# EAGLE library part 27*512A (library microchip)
CMOS EPROM 512 K (64 K x 8)
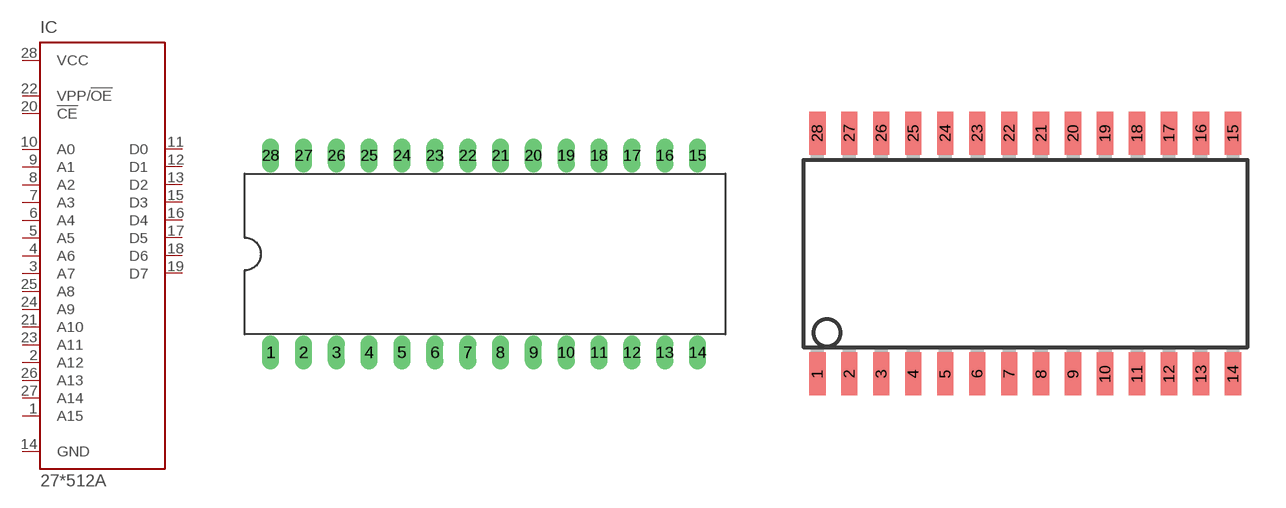
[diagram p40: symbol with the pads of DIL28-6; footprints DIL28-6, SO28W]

Designator prefix IC

## 27C512AP (MPN: M27C512-90B6; OC_FARNELL: 1642690; OC_NEWARK: 20M6389)  [DIL28-6]
1  A15  in
2  A12  in
3  A7  in
4  A6  in
5  A5  in
6  A4  in
7  A3  in
8  A2  in
9  A1  in
10  A0  in
11  D0  hiz
12  D1  hiz
13  D2  hiz
14  GND  pwr
15  D3  hiz
16  D4  hiz
17  D5  hiz
18  D6  hiz
19  D7  hiz
20  !CE  in
21  A10  in
22  VPP/!OE  in
23  A11  in
24  A9  in
25  A8  in
26  A13  in
27  A14  in
28  VCC  pwr

## 27C512ASO (OC_FARNELL: unknown; OC_NEWARK: unknown)  [SO28W]
Pads as for DIL28-6

## 27C512AL (MPN: M27C512-90C1; OC_FARNELL: 1218315; OC_NEWARK: 24M5090)  [PLCC-32]
2  A15  in
3  A12  in
4  A7  in
5  A6  in
6  A5  in
7  A4  in
8  A3  in
9  A2  in
10  A1  in
11  A0  in
13  D0  hiz
14  D1  hiz
15  D2  hiz
16  GND  pwr
18  D3  hiz
19  D4  hiz
20  D5  hiz
21  D6  hiz
22  D7  hiz
23  !CE  in
24  A10  in
25  VPP/!OE  in
27  A11  in
28  A9  in
29  A8  in
30  A13  in
31  A14  in
32  VCC  pwr

## 27C512ATS (OC_FARNELL: unknown; OC_NEWARK: unknown), 27LV512ATS (OC_FARNELL: unknown; OC_NEWARK: unknown)  [TSOP28]
1  VPP/!OE  in
2  A11  in
3  A9  in
4  A8  in
5  A13  in
6  A14  in
7  VCC  pwr
8  A15  in
9  A12  in
10  A7  in
11  A6  in
12  A5  in
13  A4  in
14  A3  in
15  A2  in
16  A1  in
17  A0  in
18  D0  hiz
19  D1  hiz
20  D2  hiz
21  GND  pwr
22  D3  hiz
23  D4  hiz
24  D5  hiz
25  D6  hiz
26  D7  hiz
27  !CE  in
28  A10  in

## 27512AVS (OC_FARNELL: unknown; OC_NEWARK: unknown)  [VSOP28-8X13]
Pads as for DIL28-6

## Footprint DIL28-6 (pad centres in mm)
Dual In Line package type P
drill 0.813 long: 1 -16.51,-7.62; 2 -13.97,-7.62; 3 -11.43,-7.62; 4 -8.89,-7.62; 5 -6.35,-7.62; 6 -3.81,-7.62; 7 -1.27,-7.62; 8 1.27,-7.62; 9 3.81,-7.62; 10 6.35,-7.62; 11 8.89,-7.62; 12 11.43,-7.62; 13 13.97,-7.62; 14 16.51,-7.62; 15 16.51,7.62; 16 13.97,7.62; 17 11.43,7.62; 18 8.89,7.62; 19 6.35,7.62; 20 3.81,7.62; 21 1.27,7.62; 22 -1.27,7.62; 23 -3.81,7.62; 24 -6.35,7.62; 25 -8.89,7.62; 26 -11.43,7.62; 27 -13.97,7.62; 28 -16.51,7.62

## Footprint SO28W (pad centres in mm)
28-Lead Plastic Small Outline (SO) Wide, 300 mil Body (SOIC) Source: http://ww1.microchip.com/downloads/en/devicedoc/39632c.pdf
smd 0.65 x 1.7: 1 -7.62,-4.78; 2 -6.35,-4.78; 3 -5.08,-4.78; 4 -3.81,-4.78; 5 -2.54,-4.78; 6 -1.27,-4.78; 7 0,-4.78; 8 1.27,-4.78; 9 2.54,-4.78; 10 3.81,-4.78; 11 5.08,-4.78; 12 6.35,-4.78; 13 7.62,-4.78; 14 8.89,-4.78; 15 8.89,4.78; 16 7.62,4.78; 17 6.35,4.78; 18 5.08,4.78; 19 3.81,4.78; 20 2.54,4.78; 21 1.27,4.78; 22 0,4.78; 23 -1.27,4.78; 24 -2.54,4.78; 25 -3.81,4.78; 26 -5.08,4.78; 27 -6.35,4.78; 28 -7.62,4.78

## Footprint PLCC-32 (pad centres in mm)
PLASTIC LEADED CHIP CARRIER rectangle, package type L
smd 2.2 x 0.6: 1 -6.83,0; 2 -6.83,-1.27; 3 -6.83,-2.54; 4 -6.83,-3.81; 14 6.83,-3.81; 15 6.83,-2.54; 16 6.83,-1.27; 17 6.83,0; 18 6.83,1.27; 19 6.83,2.54; 20 6.83,3.81; 30 -6.83,3.81; 31 -6.83,2.54; 32 -6.83,1.27
smd 0.6 x 2.2: 5 -5.08,-5.56; 6 -3.81,-5.56; 7 -2.54,-5.56; 8 -1.27,-5.56; 9 0,-5.56; 10 1.27,-5.56; 11 2.54,-5.56; 12 3.81,-5.56; 13 5.08,-5.56; 21 5.08,5.56; 22 3.81,5.56; 23 2.54,5.56; 24 1.27,5.56; 25 0,5.56; 26 -1.27,5.56; 27 -2.54,5.56; 28 -3.81,5.56; 29 -5.08,5.56

## Footprint TSOP28 (pad centres in mm)
Thin Small Outline Package Gull Wing type I, package type TS
smd 0.3 x 1: 1 -3.75,-9.7; 2 -3.25,-9.7; 3 -2.75,-9.7; 4 -2.25,-9.7; 5 -1.75,-9.7; 6 -1.25,-9.7; 7 -0.75,-9.7; 8 0.75,-9.7; 9 1.25,-9.7; 10 1.75,-9.7; 11 2.25,-9.7; 12 2.75,-9.7; 13 3.25,-9.7; 14 3.75,-9.7; 15 3.75,9.7; 16 3.25,9.7; 17 2.75,9.7; 18 2.25,9.7; 19 1.75,9.7; 20 1.25,9.7; 21 0.75,9.7; 22 -0.75,9.7; 23 -1.25,9.7; 24 -1.75,9.7; 25 -2.25,9.7; 26 -2.75,9.7; 27 -3.25,9.7; 28 -3.75,9.7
